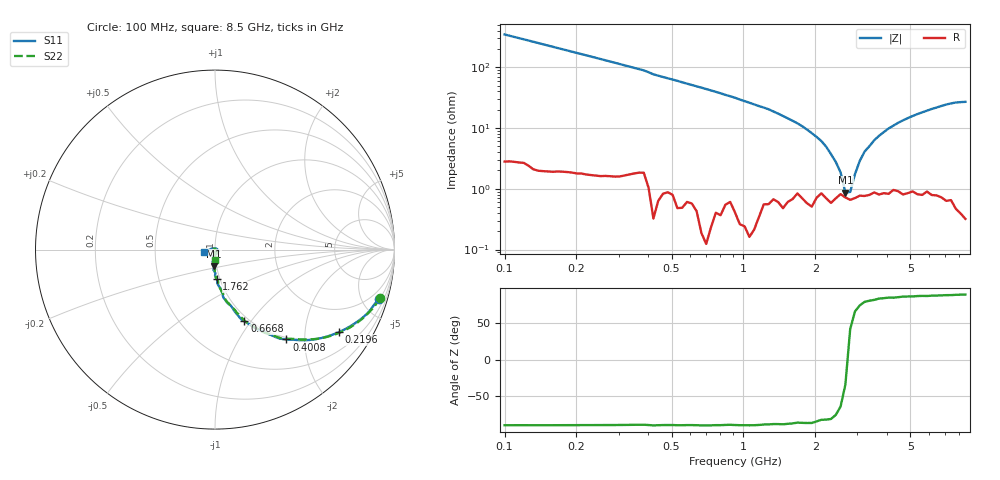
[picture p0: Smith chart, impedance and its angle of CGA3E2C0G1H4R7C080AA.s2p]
! S-parameter Generated by TDK Corporation
! Copyright(C) 2015 TDK Corporation.
! All Rights Reserved.
! TDK P/N: CGA3E2C0G1H4R7C080AA (Multilayer Ceramic Chip Capacitors)
! Property: C=4.7pF
! Size(LxWxT): 1.6x0.8x0.8mm, 0.063x0.031x0.031inches
! Model Type: s2p (Touchstone File Format Version 1.0)
! Frequency: DC=Yes Start=100MHz Stop=8500MHz 98points Log-sweep
! Note:
! Model Generated on Jun. 23, 2015
! Hash(MD5):
! Port Assignments:
!  1 ---| |--- 2
! Applicable Conditions:
!  Temperature = 25 degC
!  DC Bias Voltage = 0 V
!  Small Signal Operation
! Terms and conditions regarding TDK Simulation Models
! (1)This simulation model is being provided solely for informational purposes. Please refer to the specifications of the products in terms of detailed characteristics of such products.
! (2)In no event shall TDK Corporation of any of its subsidiaries be liable for any loss or damage arising, directly or indirectly,
!  From any information contained in this simulation model, including, but not limited to loss or damages arising from any inaccuracies, omissions or errors in connection with such information.
! (3)Any and all copyrights on this simulation model are owned by TDK Corporation.
!  Duplication or redistribution of this simulation model without prior written permission from TDK Corporation is prohibited.
! (4)This simulation model is subject to any modification or change without any prior notice.
! (5)Neither TDK Corporation nor any of its subsidiaries shall make any warranty, express or implied,
!  Including but not limited to the correctness, implied warranties of merchantability and fitness for a particular purpose with respect to this simulation models.
! (6)The use of this simulation model shall be deemed to have consented to the terms and conditions hereof.
# MHz S MA R 50
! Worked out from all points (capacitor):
!   97 points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, 100 MHz to 8.5 GHz, reference 50 ohm
!   read as one part in series: C = 4.6 pF near 100 MHz
!   lowest |Z| = 865 mohm at 2.673 GHz (marker M1)
!   series resonance near 2.729 GHz, so ESL is about 740 pH
!   S11 on the Smith chart (normalised r, x): 100 MHz: 1.12, -6.64; 219.6 MHz: 1.02, -3.00; 400.8 MHz: 0.96, -1.63; 666.8 MHz: 0.95, -0.93; 1.762 GHz: 0.97, -0.33; 8.5 GHz: 0.89, -0.02
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100  0.9526 -16.7  0.2763 73.0  0.276 73.2  0.9589 -16.5
219.618  0.8304 -33.6  0.5295 56.2  0.5288 56.5  0.8406 -33.0
400.8145  0.6393 -51.5  0.7592 38.1  0.7581 38.4  0.6387 -51.1
666.8416  0.4318 -67.7  0.8931 23.1  0.8919 23.4  0.4351 -67.0
965.6229  0.3098 -76.4  0.9462 14.2  0.9446 14.4  0.3124 -75.3
1533.871  0.194 -85.3  0.9707 4.9  0.9692 5.1  0.1922 -84.5
1762.313  0.1641 -86.6  0.9766 2.3  0.9752 2.6  0.167 -86.4
2672.798  0.09337 -94.9  0.9842 -5.1  0.9826 -4.9  0.09784 -92.4
2931.989  0.08334 -98.6  0.9849 -7.0  0.9832 -6.6  0.08673 -92.5
3870.357  0.04249 -101.1  0.9861 -12.5  0.984 -12.1  0.04169 -93.4
4245.68  0.03002 -95.5  0.986 -14.5  0.9849 -14.2  0.02948 -89.7
4446.777  0.02052 -87.0  0.9852 -15.6  0.9848 -15.2  0.02452 -99.1
4877.997  0.01769 -68.5  0.9867 -18.0  0.9846 -17.3  0.01193 -114.2
5109.044  0.019 -48.6  0.986 -19.0  0.9853 -18.7  0.01038 -142.3
5604.487  0.01867 -34.9  0.9858 -21.7  0.9839 -21.2  0.01221 177.4
5869.945  0.02169 -25.1  0.9864 -22.9  0.9837 -22.6  0.01159 169.1
6147.976  0.02025 -13.8  0.9843 -24.5  0.9848 -24.0  0.013 166.7
6744.168  0.01342 7.1  0.9856 -27.4  0.9837 -26.9  0.006464 133.8
7063.606  0.008572 47.7  0.9857 -28.9  0.9832 -28.5  0.004876 75.2
7398.175  0.00758 108.6  0.9855 -30.5  0.9837 -30.2  0.00801 -24.8
8115.603  0.03529 -175.9  0.9843 -34.1  0.9847 -33.5  0.03519 -79.7
8500  0.06052 -169.2  0.9824 -36.1  0.9818 -35.3  0.05917 -89.2
